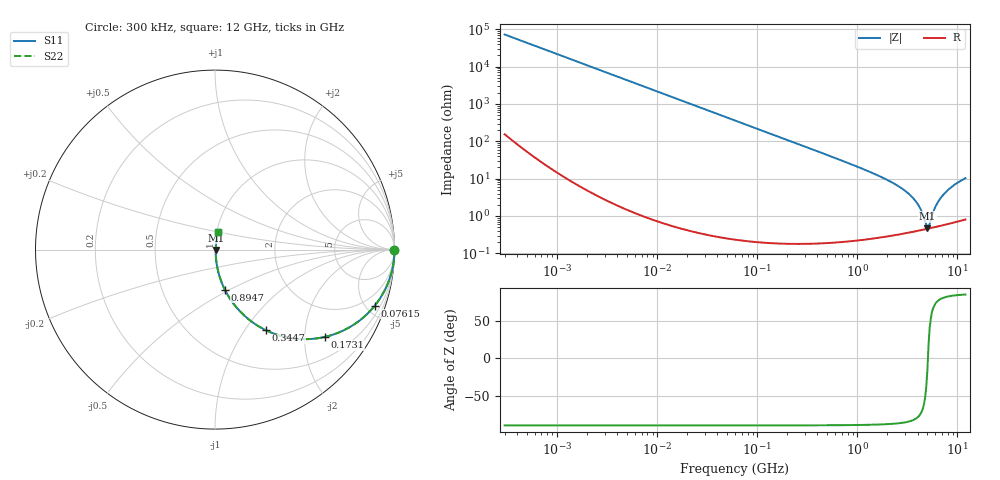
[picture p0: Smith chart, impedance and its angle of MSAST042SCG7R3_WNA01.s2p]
! MSAST042SCG7R3_WNA01  S-PARAMETER MODEL  ( General Type )
! Model Generated by TAIYO YUDEN Corporation (http://www.ty-top.com)
! Version 1.0
! TAIYO YUDEN Control No. 150820
! Copyright(c) 2015 TAIYO YUDEN CO.,LTD. All Rights Reserved.
! Product Description (link to TY-COMPAS)
! https://ds.yuden.co.jp/TYCOMPAS/or/detail?pn=MSAST042SCG7R3BWNA01&u=M
! Products Name : Multilayer Ceramic Capacitors
! Characteristics :
!  Capacitance : 7.3 pF , Rated Voltage : 25V , TCC : CG / C0G
!  Case Size : 0.4 x 0.2 / 0.016 x 0.008 [mm/inch] , Thickness : 0.2 / 0.008 [mm/inch]
!  (Conditions: Temperature = 25 degC , DC Bias Current/Voltage = 0A / 0V)
! External Node Assignments :
!  1  o---| |---o  2
! GND o---------o GND
! Frequency Range : 0.3MHz  -  12000MHz  [ 401 STEP ]
# MHz S RI R 50
! Freq[MHz].  S11 Real  S11 Imag  S21 Real  S21 Imag  S12 Real  S12 Imag  S22 Real  S22 Imag
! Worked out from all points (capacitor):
!   401 points, 300 kHz to 12 GHz, reference 50 ohm
!   read as one part in series: C = 7.31 pF near 316.3 kHz
!   lowest |Z| = 474 mohm at 5.006 GHz (marker M1)
!   series resonance near 5.071 GHz, so ESL is about 130 pH
!   S11 on the Smith chart (normalised r, x): 300 kHz: open; 76.15 MHz: 1.00, -5.71; 173.1 MHz: 1.00, -2.51; 344.7 MHz: 1.00, -1.26; 894.7 MHz: 1.00, -0.47; 12 GHz: 1.02, +0.21
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0.3  1 -0.00138  4.84e-06 0.00138  4.84e-06 0.00138  1 -0.00138
1.769972  0.9999 -0.00813  7e-05 0.00813  7e-05 0.00813  0.9999 -0.00813
10.44266  0.9977 -0.0479  0.00231 0.0479  0.00231 0.0479  0.9977 -0.0479
27.10171  0.9847 -0.1226  0.0153 0.1226  0.0153 0.1226  0.9847 -0.1226
60  0.9292 -0.2562  0.0708 0.2562  0.0708 0.2562  0.9292 -0.2562
76.15486  0.8906 -0.3117  0.1094 0.3117  0.1094 0.3117  0.8906 -0.3117
173.124  0.6117 -0.4866  0.3883 0.4866  0.3883 0.4866  0.6117 -0.4866
344.7396  0.2836 -0.4493  0.7164 0.4493  0.7164 0.4493  0.2836 -0.4493
353.9943  0.2729 -0.444  0.7271 0.444  0.7271 0.444  0.2729 -0.444
540.8523  0.1378 -0.3423  0.8622 0.3423  0.8622 0.3423  0.1378 -0.3423
894.6982  0.0544 -0.2224  0.9456 0.2224  0.9456 0.2224  0.0544 -0.2224
2088.533  0.0103 -0.0855  0.9897 0.0855  0.9897 0.0855  0.0103 -0.0855
2870.14  0.00599 -0.0512  0.994 0.0512  0.994 0.0512  0.00599 -0.0512
3642.919  0.00463 -0.0288  0.9954 0.0288  0.9954 0.0288  0.00463 -0.0288
4158.869  0.00437 -0.0172  0.9956 0.0172  0.9956 0.0172  0.00437 -0.0172
4875.354  0.00447 -0.00355  0.9955 0.00355  0.9955 0.00355  0.00447 -0.00355
5006.236  0.00453 -0.00133  0.9955 0.00133  0.9955 0.00133  0.00453 -0.00133
5278.635  0.00469 0.00408  0.9953 -0.00408  0.9953 -0.00408  0.00469 0.00408
6188.031  0.00553 0.0196  0.9945 -0.0196  0.9945 -0.0196  0.00553 0.0196
7064.448  0.00672 0.0335  0.9933 -0.0335  0.9933 -0.0335  0.00672 0.0335
8966.534  0.0104 0.0622  0.9896 -0.0622  0.9896 -0.0622  0.0104 0.0622
12000  0.0182 0.1002  0.9818 -0.1002  0.9818 -0.1002  0.0182 0.1002
